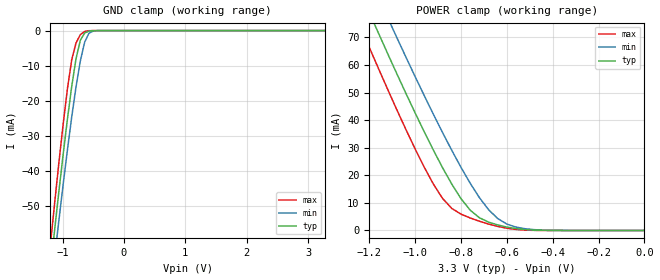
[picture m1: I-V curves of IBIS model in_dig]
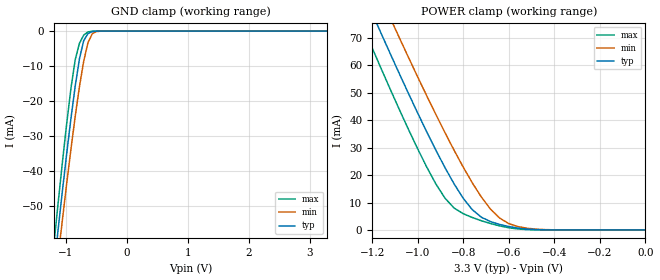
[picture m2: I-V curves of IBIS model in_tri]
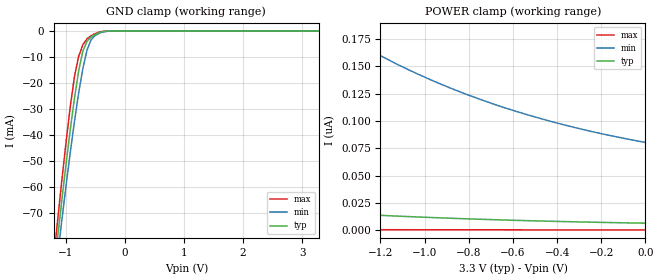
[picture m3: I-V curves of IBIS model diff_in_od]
| Integrated Devices Technolgy, Inc
[Ibis Ver]   4.1
[File Name]   9zxl1232e.ibs
[File Rev]   1.0
[Date]   Wednesday, January 24, 2018
[Source]   Integrated Devices Technolgy, Inc.
[Notes]   Rev 1.0 created by EvK
[Disclaimer] Integrated Device Technology, Inc. ("IDT") hereby grants the
   user of this IBIS model a non-exclusive, nontransferable
   license to use this IBIS model under the following terms. The
   user is granted this license only to use the IBIS model and is
   not granted rights to sell, copy (except as needed to run the
   IBIS model), rent, lease or sub-license the IBIS model in
   whole or in part, or in modified form to anyone. The User may
   modify the IBIS model to suit its specific applications, but
   rights to derivative works and such modifications shall belong
   to IDT. This IBIS model is provided on an AS IS" basis and IDT
   makes absolutely no warranty with respect to the information
   contained herein. IDT DISCLAIMS AND CUSTOMER WAIVES ALL
   WARRANTIES, EXPRESS AND IMPLIED, INCLUDING WARRANTIES OF
   MERCHANTABILITY AND FITNESS FOR A PARTICULAR PURPOSE. THE
   ENTIRE RISK AS TO QUALITY AND PERFORMANCE IS WITH THE USER
   ACCORDINGLY, IN NO EVENT SHALL IDT BE LIABLE FOR ANY DIRECT OR
   INDIRECT DAMAGES, WHETHER IN CONTRACT OR TORT, INCLUDING ANY
   LOST PROFITS OR OTHER INCIDENTAL, CONSEQUENTIAL, EXEMPLARY, OR
   PUNITIVE DAMAGES ARISING OUT OF THE USE OR APPLICATION OF THE
   IBIS model. Further, IDT reserves the right to make changes
   without notice to any product herein to improve reliability,
   function, or design. IDT does not convey any license under
   patent rights or any other intellectual property rights,
   including those of third parties. IDT is not obligated to
   provide maintenance or support for the licensed IBIS model.
   (C) Copyright Integrated Device Technology, Inc. 2016 All
   rights reserved
|   COMPONENT: 9zxl1232e
[Component]   9zxl1232e
[Manufacturer]   Integrated Device Technology, Inc.
[Package]
| variable   typ   min   max
R_pkg   81.10m   62.20m   100.00m
L_pkg   6.70nH   4.90nH   8.50nH
C_pkg   0.53pF   0.21pF   0.85pF
[Pin]   signal_name   model_name   R_pin   L_pin   C_pin
1   VDDA   POWER
2   GNDA   GND
3   SMB_WRTLOCK   in_dig
4   100M_133M#   in_dig
5   HBW_BYP_LOBW#  in_tri
6   CKPWRGD_PD   in_dig
7   GND   GND
8   VDDR   POWER
9   DIF_IN   diff_in_od
10   DIF_IN#   diff_in_od
11   SADR0_TRI   in_tri_od
12   SMBDAT   sda_od
13   SMBCLK   scl_od
14   SADR1_TRI   in_tri_od
15   FBOUT_NC#   NC
16   FBOUT_NC   NC
17   DIF_0   diff_out
18   DIF_0#   diff_out
19   OE_0#   in_dig
20   OE_1#   in_dig
21   DIF_1   diff_out
22   DIF_1#   diff_out
23   GND   GND
24   VDD   POWER
25   VDDIO   POWER
26   DIF_2   diff_out
27   DIF_2#   diff_out
28   OE_2#   in_dig
29   OE_3#   in_dig
30   DIF_3   diff_out
31   DIF_3#   diff_out
32   VDDIO   POWER
33   GND   GND
34   DIF_4   diff_out
35   DIF_4#   diff_out
36   OE_4#   in_dig
37   OE_5#   in_dig
38   DIF_5   diff_out
39   DIF_5#   diff_out
40   VDD   POWER
41   GND   GND
42   DIF_6   diff_out
43   DIF_6#   diff_out
44   OE_6#   in_dig
45   OE_7#   in_dig
46   DIF_7   diff_out
47   DIF_7#   diff_out
48   GND   GND
49   VDDIO   POWER
50   DIF_8   diff_out
51   DIF_8#   diff_out
52   OE_8#   in_dig
53   OE_9#   in_dig
54   DIF_9   diff_out
55   DIF_9#   diff_out
56   VDDIO   POWER
57   VDD   POWER
58   GND   GND
59   DIF_10   diff_out
60   DIF_10#   diff_out
61   OE_10#   in_dig
62   OE_11#   in_dig
63   DIF_11   diff_out
64   DIF_11#   diff_out
65   EPAD   GND
[Diff Pin]   inv_pin   vdiff   tdelay_typ
9   10   NA   NA
17   18   NA   NA
21   22   NA   NA
26   27   NA   NA
30   31   NA   NA
34   35   NA   NA
38   39   NA   NA
42   43   NA   NA
46   47   NA   NA
50   51   NA   NA
54   55   NA   NA
59   60   NA   NA
63   64   NA   NA
| Models and submodels in the file (7): in_dig (Input), in_tri (Input), diff_in_od (Input), in_tri_od (Input), sda_od (I/O_open_drain), scl_od (Input), diff_out (Output)
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|   Model in_dig
[Model]  in_dig
Model_type Input
Polarity   Non-Inverting
Vinl =   0.8000V
Vinh =   2.0000V
C_comp   2.1000pF   2.1000pF   2.1000pF
[Temperature Range]   25.0000   85.0000   -40.0000
[Voltage Range]   3.3000V   3.1350V   3.4650V
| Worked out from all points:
|   GND clamp passes 1 mA (typ) near -0.65 V on its own axis
|   POWER clamp passes 1 mA (typ) near -0.58 V on its own axis
[GND_clamp]
|Voltage   I(typ)   I(min)   I(max)
-3.3V     -444.4mA   -436.3mA   -455.2mA
-1.2V     -68.37mA   -75.7mA    -61.37mA
-1.13V    -56.99mA   -64.8mA    -49.35mA
-1.06V    -45.92mA   -54.16mA   -37.72mA
-920mV    -25.14mA   -33.91mA   -16.51mA
-850mV    -15.84mA   -24.53mA   -8.255mA
-780mV    -7.95mA    -15.96mA   -3.499mA
-710mV    -2.728mA   -8.626mA   -1.156mA
-640mV    -697.7uA   -3.286mA   -240.6uA
-570mV    -146.6uA   -751uA     -34.01uA
-430mV    -3.844uA   -23.08uA   -279.3nA
3.28V     213.4pA    44.16nA    205.9pA
[POWER_clamp]
|Voltage   I(typ)   I(min)   I(max)
-3.28V    509.3mA    515.8mA    504.9mA
-1.24V    86.61mA    99.33mA    74.1mA
-1.16V    71.55mA    84.5mA     58.72mA
-1.12V    64.14mA    77.19mA    51.18mA
-1.08V    56.84mA    69.96mA    43.78mA
-960mV    35.71mA    48.84mA    22.88mA
-880mV    22.69mA    35.43mA    11.57mA
-840mV    16.77mA    29.02mA    7.979mA
-760mV    7.367mA    17.14mA    4.53mA
-640mV    2.005mA    4.321mA    1.477mA
-480mV    131.2uA    293.3uA    37.64uA
0V        220.8pA    394.5pA    228.5pA
|   Model in_tri
[Model]  in_tri
Model_type Input
Polarity   Non-Inverting
Vinl =   0.8000V
Vinh =   2.0000V
C_comp   2.1400pF   2.1400pF   2.1400pF
[Temperature Range]   25.0000   85.0000   -40.0000
[Voltage Range]   3.3000V   3.1350V   3.4650V
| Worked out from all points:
|   GND clamp passes 1 mA (typ) near -0.65 V on its own axis
|   POWER clamp passes 1 mA (typ) near -0.58 V on its own axis
[GND_clamp]
|Voltage   I(typ)   I(min)   I(max)
-3.3V     -444.4mA   -436.3mA   -455.2mA
-1.2V     -68.37mA   -75.7mA    -61.37mA
-1.13V    -56.99mA   -64.8mA    -49.35mA
-1.06V    -45.92mA   -54.16mA   -37.72mA
-920mV    -25.14mA   -33.91mA   -16.51mA
-850mV    -15.84mA   -24.53mA   -8.255mA
-780mV    -7.95mA    -15.96mA   -3.499mA
-710mV    -2.728mA   -8.625mA   -1.156mA
-640mV    -697.7uA   -3.286mA   -240.6uA
-570mV    -146.6uA   -751uA     -34.01uA
-430mV    -3.844uA   -23.08uA   -279.3nA
3.28V     213.4pA    44.16nA    205.9pA
[POWER_clamp]
|Voltage   I(typ)   I(min)   I(max)
-3.28V    509.3mA    515.8mA    504.9mA
-1.24V    86.61mA    99.33mA    74.1mA
-1.16V    71.55mA    84.5mA     58.72mA
-1.12V    64.14mA    77.19mA    51.18mA
-1.08V    56.84mA    69.96mA    43.78mA
-960mV    35.71mA    48.84mA    22.88mA
-880mV    22.69mA    35.43mA    11.57mA
-840mV    16.77mA    29.02mA    7.979mA
-760mV    7.367mA    17.14mA    4.53mA
-640mV    2.005mA    4.321mA    1.477mA
-480mV    131.2uA    293.3uA    37.64uA
0V        220.8pA    394.5pA    228.4pA
|   Model diff_in_od
[Model]  diff_in_od
Model_type Input
Polarity   Non-Inverting
Vinl =   0.3000V
Vinh =   0.5000V
C_comp   3.5000pF   3.5000pF   3.5000pF
[Temperature Range]   25.0000   85.0000   -40.0000
[Voltage Range]   3.3000V   3.1350V   3.4650V
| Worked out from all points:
|   GND clamp passes 1 mA (typ) near -0.47 V on its own axis
[GND_clamp]
|Voltage   I(typ)   I(min)   I(max)
-3.3V     -581.4mA   -566.8mA   -600.3mA
-1.2V     -92.9mA    -99.3mA    -87.17mA
-1.13V    -78.34mA   -85.45mA   -71.6mA
-1.06V    -64.19mA   -71.96mA   -56.52mA
-920mV    -37.64mA   -46.39mA   -28.76mA
-850mV    -25.69mA   -34.6mA    -17.37mA
-780mV    -15.32mA   -23.82mA   -9.726mA
-710mV    -7.779mA   -14.52mA   -5.31mA
-640mV    -3.984mA   -7.427mA   -3.004mA
-500mV    -1.282mA   -1.675mA   -939.5uA
-220mV    -3.662uA   -14.35uA   -357.2nA
3.28V     6.54nA     86.14nA    391.5pA
[POWER_clamp]
|Voltage   I(typ)   I(min)   I(max)
-3.28V    57.48nA    654.6nA    1.522nA
-2.84V    43.19nA    492.3nA    1.256nA
-2.4V     32.05nA    365.8nA    1.04nA
-1.92V    22.9nA     262.2nA    852pA
-1.4V     15.85nA    182.8nA    693.7pA
-1.12V    13.05nA    151.5nA    623.8pA
-960mV    11.71nA    136.6nA    587.9pA
-800mV    10.54nA    123.6nA    554.6pA
-640mV    9.52nA     112.3nA    523.5pA
-440mV    8.427nA    100.3nA    487.7pA
-240mV    7.511nA    90.3nA     454.6pA
0V        6.607nA    80.43nA    417.9pA
